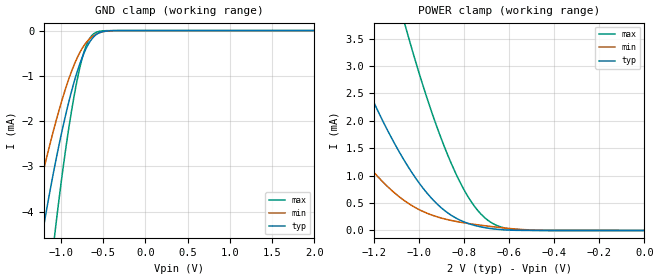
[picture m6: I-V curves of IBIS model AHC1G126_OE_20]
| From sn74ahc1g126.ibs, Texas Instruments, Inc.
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[Model]   AHC1G126_OE_20
Model_type  Input
Vinl=0.5
Vinh=1.5
| variable   typ   min   max
C_comp   2.95pF   2.48pF   3.17pF
[Temperature Range]   40   100   -40
| Ambient temperature   25   85   -40
[Voltage range]   2   2   2
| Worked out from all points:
|   GND clamp passes 1 mA (typ) near -0.82 V on its own axis
|   POWER clamp passes 1 mA (typ) near -1.02 V on its own axis
[GND Clamp]
| AHC1G126_OE_20
|   Voltage   I(typ)   I(min)   I(max)
-2V       -15.54mA   -10.83mA   -25.02mA
-1.38V    -6.369mA   -4.535mA   -10.17mA
-1.36V    -6.122mA   -4.36mA    -9.76mA
-1.22V    -4.495mA   -3.196mA   -7.031mA
-1.2V     -4.277mA   -3.039mA   -6.665mA
-1.07V    -2.961mA   -2.08mA    -4.453mA
-935mV    -1.79mA    -1.224mA   -2.506mA
-810mV    -923.9uA   -611.5uA   -1.112mA
-705mV    -406.5uA   -274.6uA   -353.7uA
-600mV    -115.8uA   -96.74uA   -55.88uA
-385mV    -2.171uA   -2.811uA   -254.8nA
2V        142.1pA    583.4pA    2.536pA
[POWER Clamp]
| AHC1G126_OE_20
|   Voltage   I(typ)   I(min)   I(max)
-2V       12.67mA    7.242mA    24.62mA
-1.6V     6.742mA    3.612mA    14.28mA
-1.335V   3.625mA    1.777mA    8.507mA
-1.2V     2.33mA     1.058mA    5.982mA
-1.065V   1.272mA    543.8uA    3.791mA
-1.05V    1.172mA    501.4uA    3.571mA
-965mV    683.1uA    315.2uA    2.418mA
-865mV    298.5uA    190uA      1.299mA
-785mV    132.1uA    129.9uA    631.8uA
-710mV    53.03uA    87.3uA     237.8uA
-565mV    2.679uA    24.45uA    12.95uA
-20.5fV   142.1pA    583.4pA    2.536pA
